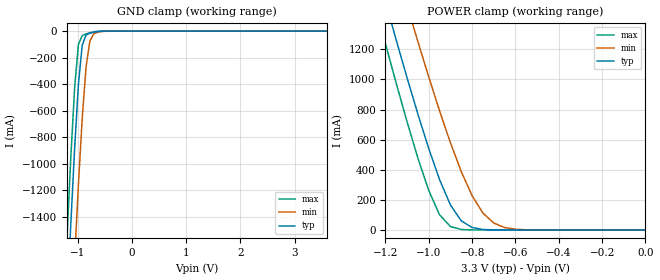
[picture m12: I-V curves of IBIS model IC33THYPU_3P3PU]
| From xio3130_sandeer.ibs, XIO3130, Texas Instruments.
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|   Model IC33THYPU_3P3PU
[Model]   IC33THYPU_3P3PU
Model_type   Input
Polarity   Non-Inverting
Vinh = 2.31V
Vinl = 0.99V
|   typ   min   max
C_comp   1.73928pF   1.8860pF   1.6401pF
[Model Spec]
|   typ   min   max
Vinh   2.31V   2.10V   2.52V
Vinl   0.99V   0.90V   1.08V
[Temperature Range]   25   125   -40
[Voltage Range]   3.30V   3.00V   3.60V
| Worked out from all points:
|   GND clamp passes 1 mA (typ) near -0.54 V on its own axis
|   POWER clamp passes 1 mA (typ) near -0.71 V on its own axis
| (Vdd votage range)   1.50V   1.35V   1.65V
| (Process strength)   nominal   weak   strong
[GND_clamp]
| voltage   I(typ)   I(min)   I(max)
-3.3V     -22.44A    -23.22A    -22A
-1.2V     -2.056A    -2.93A     -1.544A
-1.13V    -1.448A    -2.312A    -946.6mA
-1.06V    -880.3mA   -1.716A    -422.1mA
-990mV    -397.7mA   -1.154A    -99.01mA
-920mV    -105.6mA   -654.7mA   -33.8mA
-850mV    -30.2mA    -272.5mA   -21.22mA
-780mV    -16.13mA   -76.15mA   -12.33mA
-710mV    -8.988mA   -21.73mA   -5.647mA
-640mV    -4.082mA   -8.948mA   -1.809mA
-360mV    -113.4uA   -170.8uA   -163.9uA
3.6V      0A         18uA       0A
[POWER_clamp]
| voltage   I(typ)   I(min)   I(max)
-3.3V     13.18A     13.26A     13.32A
-1.25V    1.778A     2.241A     1.508A
-1.2V     1.518A     1.988A     1.238A
-1.15V    1.262A     1.738A     974.1mA
-1.1V     1.011A     1.492A     718.6mA
-1.05V    769.2mA    1.251A     477.2mA
-950mV    334.1mA    791.5mA    100.3mA
-850mV    60.72mA    388.3mA    3.223mA
-750mV    3.255mA    112.3mA    117uA
-700mV    569.4uA    46.14mA    86.33uA
-550mV    48.85uA    1.254mA    64.95uA
0V        336pA      63.37nA    111.1pA
